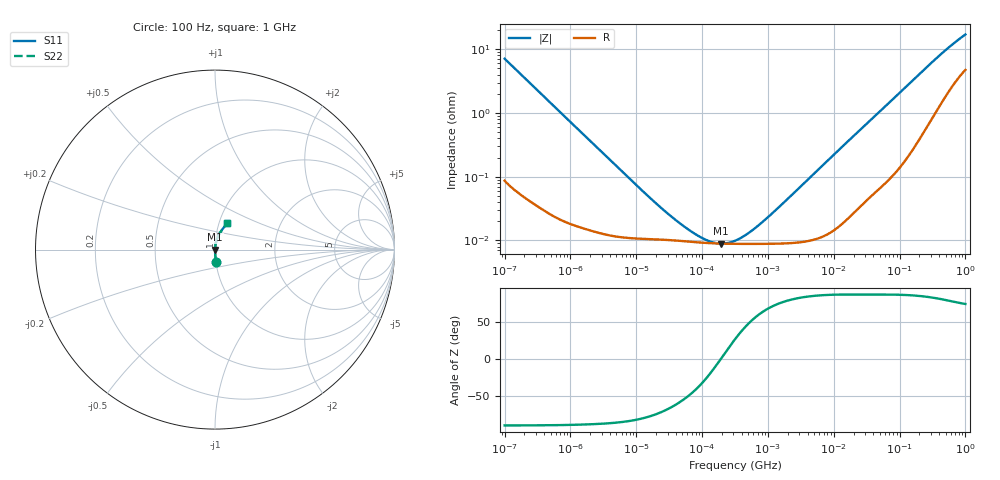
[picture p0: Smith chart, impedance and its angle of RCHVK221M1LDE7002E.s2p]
! RCHVK221M1LDE7002E  S-PARAMETER MODEL  (AEC-Q200 qualified)
! Model Generated by ELNA Corporation (http://www.ty-top.com)
! Version 1.0
! ELNA Control No.240315
! Copyright (c) 2024 ELNA CO.,LTD. All Rights Reserved.
! Products Name : CONDUCTIVE POLYMER HYBRID ALUMINUM ELECTROLYTIC CAPACITORS
! Characteristics :
!  Capacitance  :  220uF  ,  Rated voltage  :  10V
!  Operating Temp. Range  :  -55 to +125 degC  ,  Endurance  :  4000hr at 125 degC
!  Dimension D  :  6.3mm  ,  Dimension L  :  7.7mm
! Frequency Range : 100Hz - 1GHz
! External Node Assignments :
!  1  o---| |---o  2
# MHz S RI R 50
!Freq[MHz].  S11 Real  S11 Imag  S21 Real  S21 Imag  S12 Real  S12 Imag  S22 Real  S22 Imag
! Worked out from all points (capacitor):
!   401 points, 100 Hz to 1 GHz, reference 50 ohm
!   read as one part in series: C = 223 uF near 108 Hz
!   lowest |Z| = 8.93 mohm at 195 kHz (marker M1)
!   series resonance near 192.7 kHz, so ESL is about 3.1 nH
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0.0001  0.0059 -0.0708  0.9941 0.0708  0.9941 0.0708  0.0059 -0.0708
0.000113  0.00473 -0.0628  0.9953 0.0628  0.9953 0.0628  0.00473 -0.0628
0.000309  0.000885 -0.0232  0.9991 0.0232  0.9991 0.0232  0.000885 -0.0232
0.001488  0.000181 -0.00487  0.9998 0.00487  0.9998 0.00487  0.000181 -0.00487
0.009495  0.000108 -0.000772  0.9999 0.000772  0.9999 0.000772  0.000108 -0.000772
0.022131  0.000103 -0.000332  0.9999 0.000332  0.9999 0.000332  0.000103 -0.000332
0.049545  9.8e-05 -0.000145  0.9999 0.000145  0.9999 0.000145  9.8e-05 -0.000145
0.094406  9.27e-05 -6.43e-05  0.9999 6.43e-05  0.9999 6.43e-05  9.27e-05 -6.43e-05
0.110917  9.16e-05 -4.85e-05  0.9999 4.85e-05  0.9999 4.85e-05  9.16e-05 -4.85e-05
0.12517  9.09e-05 -3.73e-05  0.9999 3.73e-05  0.9999 3.73e-05  9.09e-05 -3.73e-05
0.194984  8.93e-05 1.02e-06  0.9999 -1.02e-06  0.9999 -1.02e-06  8.93e-05 1.02e-06
0.316228  8.84e-05 4.4e-05  0.9999 -4.4e-05  0.9999 -4.4e-05  8.84e-05 4.4e-05
0.356862  8.83e-05 5.6e-05  0.9999 -5.6e-05  0.9999 -5.6e-05  8.83e-05 5.6e-05
0.454465  8.82e-05 8.27e-05  0.9999 -8.27e-05  0.9999 -8.27e-05  8.82e-05 8.27e-05
0.767361  8.83e-05 0.00016  0.9999 -0.00016  0.9999 -0.00016  8.83e-05 0.00016
1.462177  8.92e-05 0.000319  0.9999 -0.000319  0.9999 -0.000319  8.92e-05 0.000319
4.704354  0.000102 0.00104  0.9999 -0.00104  0.9999 -0.00104  0.000102 0.00104
69.9842  0.00112 0.0146  0.9989 -0.0146  0.9989 -0.0146  0.00112 0.0146
176.8072  0.00443 0.0359  0.9956 -0.0359  0.9956 -0.0359  0.00443 0.0359
395.8221  0.018 0.0752  0.982 -0.0752  0.982 -0.0752  0.018 0.0752
668.3439  0.041 0.113  0.959 -0.113  0.959 -0.113  0.041 0.113
1000  0.0682 0.146  0.9318 -0.146  0.9318 -0.146  0.0682 0.146
